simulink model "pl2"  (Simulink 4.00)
settings: Solver=ode45  StartTime=0.0  StopTime=8  RelTol=1e-3
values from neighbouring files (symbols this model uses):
  m = p    (= 10)    [scr.m]    (also in Smpc.m = mp(1:max(size(mp))-1); demo1dat.m = 4; demo2dat.m = 3; essai1dat.m = 4)
  model = [y(2:ly); 1; 1; .1]    [scr.m]    (also in Smpc.m = modelpd(:,1:nu); essai2dat.m = tfd2step(1.6,delt,1,g); mynlcmpc.m = modelpd(:,1:nu); mynlcmpc2.m = modelpd(:,1:nu))
  p = 10    [scr.m]    (also in Smpc.m = mp(max(size(mp))); demo1dat.m; demo2dat.m; essai1dat.m)
  ulim = [-4 4 .5]    [scr.m]    (also in Smpc.m = [-inf*ones(1,nu) inf*ones(1,nu) 1e6*ones(1,nu)]; essai2dat.m = [-5 40 3]; mynlcmpc.m = [-inf*ones(1,nu) inf*ones(1,nu) 1e6*ones(1,nu)]; mynlcmpc2.m = [-inf*ones(1,nu) inf*ones(1,nu) 1e6*ones(1,nu)])
  uwt = 1    [scr.m]    (also in Smpc.m = yuwt(:,ny+1:ny+nu); demo1dat.m = [0 0]; demo2dat.m = 0.6*[1 1]; essai1dat.m = [0 0])
  ylim = [-inf inf]    [scr.m]    (also in Smpc.m = [ylim; ylim(N,:)]; essai2dat.m = [-40 40]; mynlcmpc.m = [ylim; ylim(N,:)]; mynlcmpc2.m = [ylim; ylim(N,:)])
  ywt = 5    [scr.m]    (also in Smpc.m = yuwt(:,1:ny); demo1dat.m = [1 1]; demo2dat.m = [0.2,0,1]; essai1dat.m = [1 1])

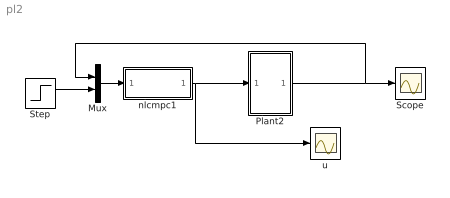
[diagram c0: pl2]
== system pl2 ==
  Mux : Mux  Inputs=2
  Plant2 : Subsystem
  Scope : Scope
  Step : Step  Time=1  Before=0  After=1  SampleTime=0
  nlcmpc1 : Subsystem  AncestorBlock=nlmpclib/nlcmpc  mask(Smpc){modelpd=[model []], yuwt=[ywt uwt], mp=[m p], yulim=[ylim ulim], tfilter=[], ud0=[0 []]}
      mask help: Masked MATLAB function block calls nlcmpc, links CMPC and SIMULINK.
  u : Scope
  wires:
  Plant2/1(y) -> Scope/1, Mux/1
  nlcmpc1/1(Out1) -> u/1, Plant2/1(u)
  Mux/1 -> nlcmpc1/1(In1)
  Step/1 -> Mux/2

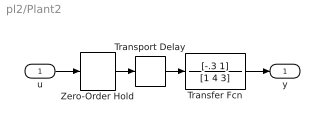
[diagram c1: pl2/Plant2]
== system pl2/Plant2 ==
  u : Inport  Port=1  LatchInput=off
  Transfer Fcn : TransferFcn  Numerator=[-.3 1]  Denominator=[1 4 3]  AbsoluteTolerance=auto  Realization=auto
  Transport Delay : TransportDelay  DelayTime=.2  InitialInput=0  BufferSize=1024  PadeOrder=0
  Zero-Order Hold : ZeroOrderHold  SampleTime=0.1
  y : Outport  Port=1
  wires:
  Zero-Order Hold/1 -> Transport Delay/1
  Transport Delay/1 -> Transfer Fcn/1
  u/1 -> Zero-Order Hold/1
  Transfer Fcn/1 -> y/1

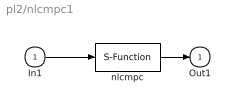
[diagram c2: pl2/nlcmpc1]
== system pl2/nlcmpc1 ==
  In1 : Inport  Port=1  LatchInput=off
  nlcmpc : S-Function  FunctionName=Smpc  Parameters=modelpd,mp,tfilter,yuwt,ud0,yulim  PortCounts=[]  SFunctionModules=''
  Out1 : Outport  Port=1  InitialOutput=0
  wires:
  In1/1 -> nlcmpc/1
  nlcmpc/1 -> Out1/1
